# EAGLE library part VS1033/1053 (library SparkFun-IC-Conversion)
VS1053B MP3 and MIDI Codec AAC/MP3/WMA/MIDI/Ogg Audio Player and Ogg Recording Device LQFP-48 7x7x1.4 mm Datasheet SparkFun Products Storefront component: MP3 and MIDI Codec - VS1053B (COM-08892) SparkFun MP3 Player Shield (DEV-12660) LilyPad MP3 (DEV-11013) SparkFun Music Instrument Shield (DEV-10587)
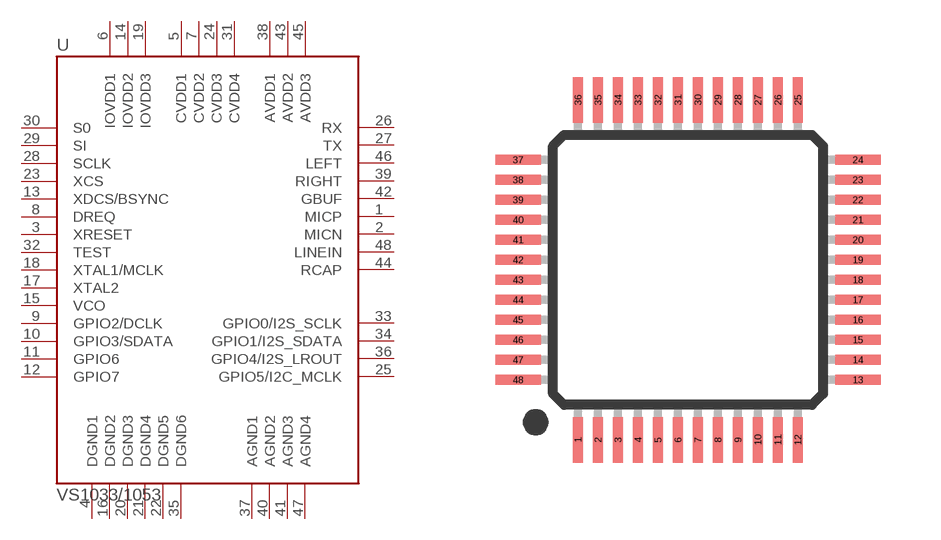
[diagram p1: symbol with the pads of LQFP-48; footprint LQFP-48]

Designator prefix U

## VS1033/1053SMD (PROD_ID: IC-12665; VALUE: VS1053B)  [LQFP-48]
1  MICP
2  MICN
3  XRESET
4  DGND1
5  CVDD1
6  IOVDD1
7  CVDD2
8  DREQ
9  GPIO2/DCLK
10  GPIO3/SDATA
11  GPIO6
12  GPIO7
13  XDCS/BSYNC
14  IOVDD2
15  VCO
16  DGND2
17  XTAL2
18  XTAL1/MCLK
19  IOVDD3
20  DGND3
21  DGND4
22  DGND5
23  XCS
24  CVDD3
25  GPIO5/I2C_MCLK
26  RX
27  TX
28  SCLK
29  SI
30  S0
31  CVDD4
32  TEST
33  GPIO0/I2S_SCLK
34  GPIO1/I2S_SDATA
35  DGND6
36  GPIO4/I2S_LROUT
37  AGND1
38  AVDD1
39  RIGHT
40  AGND2
41  AGND3
42  GBUF
43  AVDD2
44  RCAP
45  AVDD3
46  LEFT
47  AGND4
48  LINEIN

## Footprint LQFP-48 (pad centres in mm)
LQFP -48 Specifications: Pin count: 48 Example device(s): VS1000
smd 0.254 x 1.143: 1 -2.75,-4.25; 2 -2.25,-4.25; 3 -1.75,-4.25; 4 -1.25,-4.25; 5 -0.75,-4.25; 6 -0.25,-4.25; 7 0.25,-4.25; 8 0.75,-4.25; 9 1.25,-4.25; 10 1.75,-4.25; 11 2.25,-4.25; 12 2.75,-4.25; 25 2.75,4.25; 26 2.25,4.25; 27 1.75,4.25; 28 1.25,4.25; 29 0.75,4.25; 30 0.25,4.25; 31 -0.25,4.25; 32 -0.75,4.25; 33 -1.25,4.25; 34 -1.75,4.25; 35 -2.25,4.25; 36 -2.75,4.25
smd 1.143 x 0.254: 13 4.25,-2.75; 14 4.25,-2.25; 15 4.25,-1.75; 16 4.25,-1.25; 17 4.25,-0.75; 18 4.25,-0.25; 19 4.25,0.25; 20 4.25,0.75; 21 4.25,1.25; 22 4.25,1.75; 23 4.25,2.25; 24 4.25,2.75; 37 -4.25,2.75; 38 -4.25,2.25; 39 -4.25,1.75; 40 -4.25,1.25; 41 -4.25,0.75; 42 -4.25,0.25; 43 -4.25,-0.25; 44 -4.25,-0.75; 45 -4.25,-1.25; 46 -4.25,-1.75; 47 -4.25,-2.25; 48 -4.25,-2.75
